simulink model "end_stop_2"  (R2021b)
settings: Solver=VariableStepAuto  StartTime=0.0  StopTime=20  RelTol=1e-3
libraries: fl_lib x15, nesl_utility x3, sdl_lib x1

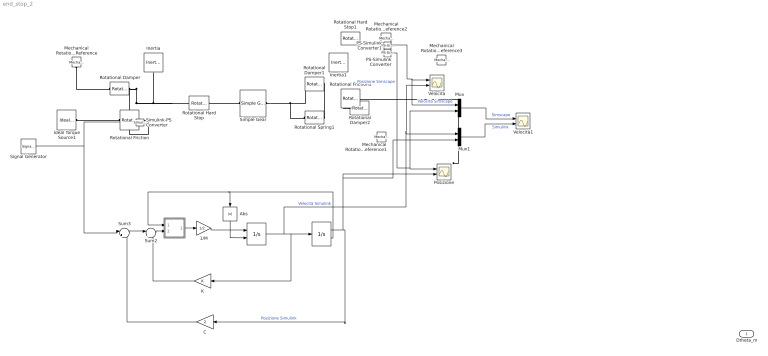
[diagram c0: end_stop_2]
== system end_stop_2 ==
  " " : Integrator  ExternalReset=rising
  "  " : Integrator  LimitOutput=on  UpperSaturationLimit=1  LowerSaturationLimit=-1  ShowSaturationPort=on
  "                       " : Subsystem
  1/M : Gain  Gain=1/2
  Abs : Abs
  C : Gain  Gain=2
  Ideal Torque Source1 : fl_lib/Mechanical/Mechanical Sources/Ideal Torque Source
  Inertia : fl_lib/Mechanical/Rotational Elements/Inertia  inertia=0.085 kg*m^2  num_ports=foundation.enum.numPorts2.one  w_specify=off  w_priority=High  w=0 rad/s  w_nominal_specify=off  w_nominal_unit=rad/s  w_nominal_value=1  t_specify=off  t_priority=None  t=0 N*m  t_nominal_specify=off  t_nominal_unit=N*m  t_nominal_value=1
  Inertia1 : fl_lib/Mechanical/Rotational Elements/Inertia  inertia=50 kg*m^2  num_ports=foundation.enum.numPorts2.one  w_specify=off  w_priority=High  w=0 rad/s  w_nominal_specify=off  w_nominal_unit=rad/s  w_nominal_value=1  t_specify=off  t_priority=None  t=0 N*m  t_nominal_specify=off  t_nominal_unit=N*m  t_nominal_value=1
  K : Gain
  Mechanical Rotational Reference{,1..3} (4 alike) : fl_lib/Mechanical/Rotational Elements/Mechanical Rotational Reference
  Mux : Mux  Inputs=2
  Mux1 : Mux  Inputs=2
  PS-Simulink Converter : nesl_utility/PS-Simulink Converter  PhysicalDomain=network_engine_domain  SubClassName=ps_output  LeftPortType=input  RightPortType=output  PseudoPeriodic=off  Frequencies=[]  Unit=inherit  AffineConversion=off
  PS-Simulink Converter1 : nesl_utility/PS-Simulink Converter  PhysicalDomain=network_engine_domain  SubClassName=ps_output  LeftPortType=input  RightPortType=output  PseudoPeriodic=off  Frequencies=[]  Unit=inherit  AffineConversion=off
  Posizione : Scope  NumInputPorts=2
  Rotational Damper : fl_lib/Mechanical/Rotational Elements/Rotational Damper  D=0.03 N*m/(rad/s)  w_specify=off  w_priority=None  w=0 rad/s  w_nominal_specify=off  w_nominal_unit=rad/s  w_nominal_value=1  t_specify=off  t_priority=None  t=0 N*m  t_nominal_specify=off  t_nominal_unit=N*m  t_nominal_value=1
  Rotational Damper1 : fl_lib/Mechanical/Rotational Elements/Rotational Damper  D=50 N*m/(rad/s)  w_specify=off  w_priority=None  w=0 rad/s  w_nominal_specify=off  w_nominal_unit=rad/s  w_nominal_value=1  t_specify=off  t_priority=None  t=0 N*m  t_nominal_specify=off  t_nominal_unit=N*m  t_nominal_value=1
  Rotational Damper2 : fl_lib/Mechanical/Rotational Elements/Rotational Damper  D=100 N*m/(rad/s)  w_specify=off  w_priority=None  w=0 rad/s  w_nominal_specify=off  w_nominal_unit=rad/s  w_nominal_value=1  t_specify=off  t_priority=None  t=0 N*m  t_nominal_specify=off  t_nominal_unit=N*m  t_nominal_value=1
  Rotational Friction : fl_lib/Mechanical/Rotational Elements/Rotational Friction  brkwy_trq=5 N*m  brkwy_vel=0.1 rad/s  Col_trq=5 N*m  visc_coef=0 N*m/(rad/s)  w_specify=off  w_priority=None  w=0 rad/s  w_nominal_specify=off  w_nominal_unit=rad/s  w_nominal_value=1  t_specify=off  t_priority=None  t=0 N*m  t_nominal_specify=off  t_nominal_unit=N*m  t_nominal_value=1
  Rotational Friction1 : fl_lib/Mechanical/Rotational Elements/Rotational Friction  brkwy_trq=500 N*m  brkwy_vel=0.1 rad/s  Col_trq=500 N*m  visc_coef=0 N*m/(rad/s)  w_specify=off  w_priority=None  w=0 rad/s  w_nominal_specify=off  w_nominal_unit=rad/s  w_nominal_value=1  t_specify=off  t_priority=None  t=0 N*m  t_nominal_specify=off  t_nominal_unit=N*m  t_nominal_value=1
  Rotational Hard Stop : fl_lib/Mechanical/Rotational Elements/Rotational Hard Stop  upper_bnd=1 deg  lower_bnd=-1 deg  stiff_up=1e6 N*m/rad  stiff_low=1e6 N*m/rad  D_up=0.01 N*m/(rad/s)  D_low=0.01 N*m/(rad/s)  model=simscape.enum.hardstop.smooth  transition=0.001 rad  w_specify=off  w_priority=None  w=0 rad/s  w_nominal_specify=off  w_nominal_unit=rad/s  w_nominal_value=1  t_specify=off  t_priority=None  t=0 N*m  t_nominal_specify=off  t_nominal_unit=N*m  t_nominal_value=1  phi_specify=off  phi_priority=High  phi=0 rad  phi_nominal_specify=off  phi_nominal_unit=rad  phi_nominal_value=1
  Rotational Hard Stop1 : fl_lib/Mechanical/Rotational Elements/Rotational Hard Stop  upper_bnd=1 rad  lower_bnd=-1 rad  stiff_up=1e6 N*m/rad  stiff_low=1e6 N*m/rad  D_up=0.01 N*m/(rad/s)  D_low=0.01 N*m/(rad/s)  model=simscape.enum.hardstop.smooth  transition=0.001 rad  w_specify=off  w_priority=None  w=0 rad/s  w_nominal_specify=off  w_nominal_unit=rad/s  w_nominal_value=1  t_specify=off  t_priority=None  t=0 N*m  t_nominal_specify=off  t_nominal_unit=N*m  t_nominal_value=1  phi_specify=off  phi_priority=High  phi=0 rad  phi_nominal_specify=off  phi_nominal_unit=rad  phi_nominal_value=1
  Rotational Spring1 : fl_lib/Mechanical/Rotational Elements/Rotational Spring  spr_rate=50 N*m/rad  w_specify=off  w_priority=None  w=0 rad/s  w_nominal_specify=off  w_nominal_unit=rad/s  w_nominal_value=1  t_specify=off  t_priority=None  t=0 N*m  t_nominal_specify=off  t_nominal_unit=N*m  t_nominal_value=1  phi_specify=off  phi_priority=High  phi=0 rad  phi_nominal_specify=off  phi_nominal_unit=rad  phi_nominal_value=1
  Signal Generator : SignalGenerator  Amplitude=100  Frequency=2  Units=rad/sec
  Simple Gear : sdl_lib/Gears/Simple Gear  ratio=100  rotation_direction=sdl.enum.shaftOutputDirection.same  friction_model=sdl.enum.gear_efficiencies_load.off  T_noload=0.1 N*m  T_nom=5 N*m  efficiency_nom=0.8  efficiency=0.8  temperature_TLU=[280, 300, 320] K  load_TLU=[1, 5, 10] N*m  efficiency_TLU=[.95, .9, .85]  efficiency_TLU2=[.85, .8, .75; .95, .9, .85; .85, .8, .7]  w_thr=0.01 rad/s  pwr_thr=0.001 W  backlash_model=sdl.enum.backlashModel.Off  backlash_distance=1e-3 mm  x0=0 mm  r_base=0.1 m  hardstop_model=simscape.enum.hardstop.smooth  transition=1e-4 mm  backlash_stiffness=1e7 N/m  backlash_damping=1e6 N/(m/s)  e=0  v_tol=0.001 m/s  mu_visc=[0, 0] N*m/(rad/s)  enable_faults=simscape.enum.onoff.off  efficiency_fault=0.05  external_fault=simscape.enum.onoff.off  temporal_fault=simscape.enum.onoff.off  fault_time=5 s  fault_angles=pi / 12 rad  report_fault=simscape.enum.assert.action.none  thermal_mass=50 J/K  temperature_specify=off  temperature_priority=High  temperature=300 K  temperature_nominal_specify=off  temperature_nominal_unit=K  temperature_nominal_value=1
  Simulink-PS Converter : nesl_utility/Simulink-PS Converter  PhysicalDomain=network_engine_domain  SubClassName=ps_input  LeftPortType=input  RightPortType=output  PseudoPeriodic=off  Frequencies=[]  NoiseDistribution=none  NoiseParameters=[]  Unit=1  AffineConversion=off  FilteringAndDerivatives=provide  SimscapeFilterOrder=1  InputFilterTimeConstant=0.001  UdotUserProvided=0
  Sum2 : Sum  Inputs=|+-
  Sum3 : Sum  Inputs=|+-
  Velocità : Scope  NumInputPorts=2
  Velocità1 : Scope  NumInputPorts=2
  Dtheta_m : Outport
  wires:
  PS-Simulink Converter1/1 -> Mux/1, Velocità/1  "Velocità Simscape"
  PS-Simulink Converter/1 -> Mux/2, Posizione/1  "Posizione Simscape"
  "                       "/1(Act) -> 1/M/1
  " "/1 -> Velocità/2, Mux1/1, K/1, "  "/1  "Velocità Simulink"
  Sum3/1 -> Sum2/1
  Sum2/1 -> "                       "/2(Act ThC)
  C/1 -> Sum3/2
  Abs/1 -> " "/2
  "  "/2 -> "                       "/1(Sat Port), Abs/1
  1/M/1 -> " "/1
  "  "/1 -> Mux1/2, Posizione/2, C/1  "Posizione Simulink"
  K/1 -> Sum2/2
  Signal Generator/1 -> Sum3/1, Simulink-PS Converter/1
  Mux/1 -> Velocità1/1  "Simscape"
  Mux1/1 -> Velocità1/2  "Simulink"
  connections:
  Rotational Damper2/LConn1 -- ?
  Rotational Damper/RConn1 -- Rotational Friction/RConn1 -- Rotational Hard Stop/LConn1 -- Inertia/LConn1
  Simple Gear/RConn1 -- Rotational Damper1/LConn1 -- Rotational Spring1/LConn1
  Ideal Torque Source1/LConn1 -- Rotational Friction/LConn1
  Rotational Hard Stop/RConn1 -- Simple Gear/LConn1
  Mechanical Rotational Reference/LConn1 -- Rotational Damper/LConn1
  Rotational Damper1/RConn1 -- Rotational Spring1/RConn1
  Rotational Friction1/LConn1 -- ?

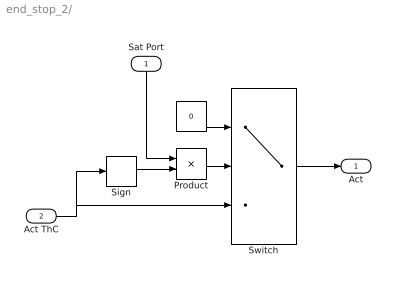
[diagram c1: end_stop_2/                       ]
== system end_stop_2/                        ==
  Sat Port : Inport
  Act ThC : Inport  Port=2
  "    " : Constant  Value=0
  Product : Product  RndMeth=Zero
  Sign : Signum
  Switch : Switch  Threshold=0.5
  Act : Outport
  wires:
  Act ThC/1 -> Switch/3, Sign/1
  Product/1 -> Switch/2
  Sign/1 -> Product/2
  "    "/1 -> Switch/1
  Switch/1 -> Act/1
  Sat Port/1 -> Product/1
